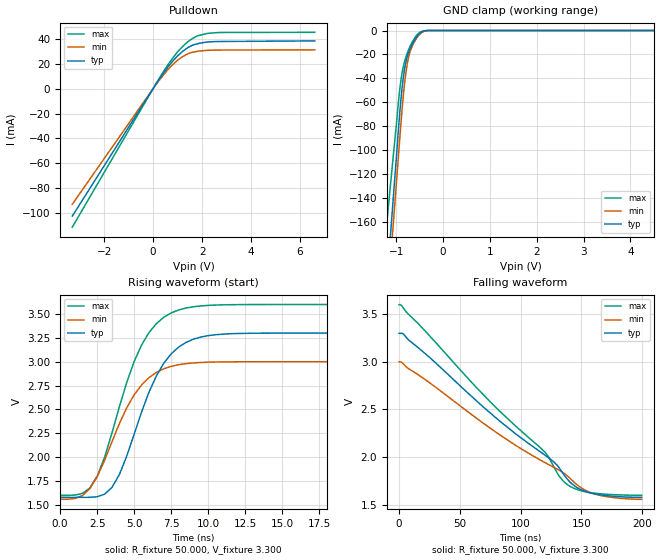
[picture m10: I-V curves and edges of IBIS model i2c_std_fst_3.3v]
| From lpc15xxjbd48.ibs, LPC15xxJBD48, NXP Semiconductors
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[Model]   i2c_std_fst_3.3v
Model_type I/O_open_drain
Vinl=9.900E-01
Vinh=2.310E+00
Vref=3.300E+00
Rref=2.000E+03
Cref=0.000E+00
Vmeas=1.650E+00
C_comp   2.020E-12   2.020E-12   2.020E-12
[Voltage Range]   3.300E+00   3.000E+00   3.600E+00
[POWER Clamp Reference]   3.300E+00   3.000E+00   3.600E+00
[GND Clamp Reference]   0.000E+00   0.000E+00   0.000E+00
[Pullup Reference]   3.300E+00   3.000E+00   3.600E+00
[Pulldown Reference]   0.000E+00   0.000E+00   0.000E+00
[Temperature Range]   25   85   -40
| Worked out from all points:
|   slope of the pulldown table from 0 to 0.495 V, typ, clamps not added: 34.6 ohm
|   GND clamp passes 1 mA (typ) near -0.45 V on its own axis
|   rising waveform, R_fixture 50.000, V_fixture 3.300: 20-80 % time 2.62ns typ, 2.63ns min, 2.59ns max; typ from 1.58 V to 3.3 V
|   falling waveform, R_fixture 50.000, V_fixture 3.300: 20-80 % time 96.5ns typ, 101ns min, 92.8ns max; typ from 3.3 V to 1.58 V
[GND Clamp]
-3.3V     -1.288A    -1.312A    -1.005A
-1.02V    -116mA     -137.9mA   -86.12mA
-940mV    -74.66mA   -96.67mA   -53.45mA
-880mV    -48.47mA   -66.8mA    -35.73mA
-840mV    -35.84mA   -49.78mA   -28.18mA
-780mV    -23.66mA   -30.76mA   -20.38mA
-720mV    -16.32mA   -19.43mA   -14.35mA
-660mV    -11.16mA   -12.88mA   -9.59mA
-560mV    -4.914mA   -5.966mA   -3.692mA
-460mV    -1.244mA   -1.762mA   -760.5uA
-320mV    0A         0A         0A
6.6V      0A         0A         0A
[Pulldown]
-3.3V     -102.3mA   -92.81mA   -111.2mA
160mV     4.868mA    4.339mA    5.348mA
580mV     16.62mA    14.63mA    18.4mA
840mV     22.82mA    19.93mA    25.49mA
1.22V     30.04mA    25.8mA     34.03mA
1.46V     33.29mA    28.19mA    38.23mA
1.84V     36.09mA    29.95mA    42.47mA
2.52V     37.67mA    30.85mA    44.78mA
6.6V      38.25mA    31.08mA    45.12mA
[Rising Waveform]
R_fixture = 50.000
V_fixture = 3.300
V_fixture_min = 3.000
V_fixture_max = 3.600
|  time   V(typ)   V(min)   V(max)
0s        1.578V     1.557V     1.599V
2ns       1.578V     1.668V     1.675V
2.5ns     1.584V     1.794V     1.799V
3.5ns     1.683V     2.161V     2.255V
4.5ns     2.013V     2.519V     2.786V
5.5ns     2.475V     2.758V     3.176V
6.5ns     2.853V     2.888V     3.4V
7.5ns     3.084V     2.952V     3.512V
11ns      3.289V     2.998V     3.596V
31ns      3.3V       3V         3.6V
[Falling Waveform]
R_fixture = 50.000
V_fixture = 3.300
V_fixture_min = 3.000
V_fixture_max = 3.600
|  time   V(typ)   V(min)   V(max)
0s        3.3V       3V         3.6V
3.5ns     3.293V     2.978V     3.564V
76.5ns    2.446V     2.29V      2.56V
120ns     2.021V     1.942V     2.053V
131.5ns   1.89V      1.863V     1.804V
137.5ns   1.782V     1.813V     1.72V
146.5ns   1.679V     1.708V     1.659V
160ns     1.616V     1.616V     1.623V
176.5ns   1.589V     1.575V     1.606V
199.5ns   1.578V     1.557V     1.599V
[Ramp]
dV/dt_r   1.0334E+00/2.5890E-09   8.6117E-01/2.5970E-09   1.2065E+00/2.5760E-09
dV/dt_f   1.0334E+00/9.6621E-08   8.6117E-01/1.0152E-07   1.2065E+00/9.2791E-08
R_load = 50
